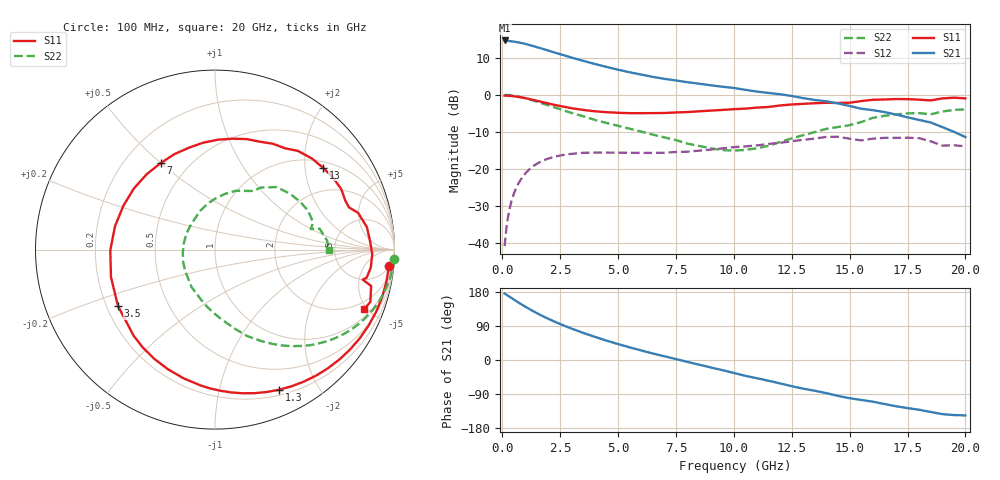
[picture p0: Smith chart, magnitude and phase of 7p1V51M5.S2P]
! Infineon Technologies  Discrete & RF Semiconductors
! bfp620
! VCE =  1.5 V,  IC =  1.5 mA
! Common Emitter S-Parameters:  Sep 2002
# GHz  S  MA  R  50
!  f  S11  S21  S12  S22
! GHz  MAG  ANG  MAG  ANG  MAG  ANG  MAG  ANG
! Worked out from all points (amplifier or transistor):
!   59 points, 100 MHz to 20 GHz, reference 50 ohm
!   highest |S21| = 14.6 dB at 100 MHz (marker M1)
!   |S21| within 3 dB of that: start of sweep to 2.131 GHz
!   unconditionally stable (mu >= 1): 6.079 GHz to 15.74 GHz; 17.62 GHz to end of sweep
!   at 1 GHz: K = 0.13, MSG = 17.4 dB, |S12| = -21.1 dB
!   at 5.5 GHz: K = 0.91, MSG = 10.8 dB, |S12| = -15.6 dB
!   at 20 GHz: K = 1.45, MAG = -2.7 dB, |S12| = -13.9 dB
!   S11 on the Smith chart (normalised r, x): 100 MHz: 5, -19; 1.3 GHz: 0.26, -1.52; 3.5 GHz: 0.25, -0.25; 7 GHz: 0.35, +0.50; 13 GHz: 1.17, +2.49; 20 GHz: 1.44, -4.80
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0.1  0.9733 -5.5  5.378 175.4  0.0092 86.8  0.9987 -3.0
0.2  0.972 -10.6  5.324 171.5  0.0186 84.2  0.9946 -6.0
0.3  0.9683 -15.8  5.278 167.5  0.0281 81.3  0.9884 -9.0
0.7  0.9359 -36.5  5.063 151.7  0.0644 68.5  0.9443 -20.3
1  0.8996 -51.4  4.825 140.5  0.0879 59.1  0.8968 -28.0
1.3  0.8582 -65.5  4.553 130.1  0.1076 50.5  0.8431 -35.0
1.8  0.7881 -87.5  4.097 114.2  0.1318 38.2  0.7524 -45.0
2.4  0.7161 -111.6  3.589 97.5  0.1502 26.2  0.6539 -54.8
3  0.6601 -133.4  3.156 82.7  0.1606 16.3  0.5698 -63.3
3.5  0.6251 -149.9  2.858 71.4  0.1658 9.4  0.5131 -69.7
4  0.5995 -165.2  2.592 61.0  0.1671 3.3  0.4594 -75.3
5  0.5721 166.9  2.175 42.0  0.1667 -5.2  0.3823 -85.9
6  0.5658 143.0  1.869 25.2  0.1654 -11.3  0.3196 -98.3
7  0.5688 122.2  1.639 9.9  0.1661 -15.1  0.267 -112.4
9  0.6127 88.4  1.343 -19.7  0.1831 -22.3  0.1906 -158.2
10.5  0.6514 67.3  1.165 -41.8  0.2022 -30.7  0.1816 152.7
12  0.718 50.0  1.017 -61.8  0.2258 -38.7  0.2322 110.5
13  0.7551 37.2  0.901 -75.7  0.2476 -46.6  0.2865 89.0
13.5  0.7698 31.5  0.851 -81.2  0.258 -51.2  0.3152 79.8
15  0.7824 17.5  0.707 -100.9  0.2566 -71.0  0.3896 56.9
17  0.8764 -1.6  0.543 -122.0  0.2634 -84.3  0.5438 29.4
20  0.8952 -21.7  0.27 -146.2  0.203 -108.9  0.6353 -0.3
